TYPE "EN_DataType"
VERSION : 0.1


  STRUCT
   UNKNOWN : BYTE ;	//Unknown data type
   TYPE_BOOL : BYTE  := B#16#1;	//8 bit boolean (0 (FALSE) … 1 (TRUE))
   TYPE_SINT : BYTE  := B#16#2;	//8 bit signed short integer (-128 … 127)
   TYPE_USINT : BYTE  := B#16#3;	//8 bit unsigned short integer (0 … 255)
   TYPE_INT : BYTE  := B#16#4;	//16 bit signed integer (-32768 … 32767)
   TYPE_UINT : BYTE  := B#16#5;	//16 bit unsigned integer (0 … 65535)
   TYPE_DINT : BYTE  := B#16#6;	//32 bit signed long integer (-2147483648 … 2147483647)
   TYPE_UDINT : BYTE  := B#16#7;	//32 bit unsigned long integer (0 … 4294967295)
   TYPE_BYTE : BYTE  := B#16#8;	//8 bit unsigned short integer (0 … 255)
   TYPE_WORD : BYTE  := B#16#9;	//16 bit unsigned integer (0 … 65535)
   TYPE_DWORD : BYTE  := B#16#A;	//32 bit unsigned long integer (0 … 4294967295)
   TYPE_REAL : BYTE  := B#16#B;	//32 bit float (1.400e-45 … 3.403e+38)
  END_STRUCT ;
END_TYPE

